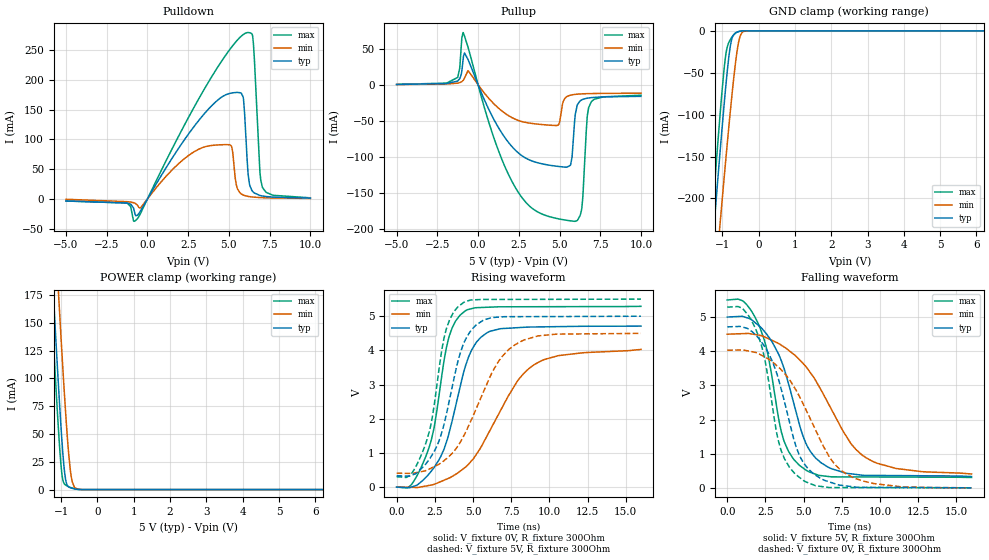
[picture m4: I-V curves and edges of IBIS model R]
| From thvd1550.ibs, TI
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|   R Model
[Model]   R
Model_type   3-state
Polarity   Non-Inverting
Vmeas = 2.5
Vref = 0
Cref = 2pF
Rref = 100000
|   typ   min   max
C_comp   6.849E-12   6.632E-12   7.073E-12
| Where Nom  PVT is Nominal Process, 5V, 27C
|   Fast PVT is Strong Process,  5.5V, -40C
|   Slow PVT is Weak Process,   4.5, 150C
[Voltage Range]   5   4.5   5.5
|Junction Temperature
[Temperature Range]   27   150   -40
[Pullup Reference]   5   4.5   5.5
[Pulldown Reference]   -0   0   0
[Power Clamp Reference]   5   4.5   5.5
[GND Clamp Reference]   0   0   0
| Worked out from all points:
|   slope of the pulldown table from 0 to 0.75 V, typ, clamps not added: 21.5 ohm
|   slope of the pullup table from 0 to 0.75 V, typ, clamps not added: 19.6 ohm
|   GND clamp passes 1 mA (typ) near -0.56 V on its own axis
|   POWER clamp passes 1 mA (typ) near -0.67 V on its own axis
|   falling waveform, V_fixture 5V, R_fixture 300Ohm: 20-80 % time 2.01ns typ, 3.35ns min, 1.42ns max; typ from 5 V to 0.332 V
|   rising waveform, V_fixture 0V, R_fixture 300Ohm: 20-80 % time 1.74ns typ, 3.15ns min, 1.29ns max; typ from 0 V to 4.71 V
|   rising waveform, V_fixture 5V, R_fixture 300Ohm: 20-80 % time 1.58ns typ, 2.64ns min, 1.21ns max; typ from 0.332 V to 5 V
|   falling waveform, V_fixture 0V, R_fixture 300Ohm: 20-80 % time 1.85ns typ, 2.86ns min, 1.37ns max; typ from 4.71 V to 0 V
[Pulldown]
|   Voltage   I(typ)   I(min)   I(max)
-5V       -3.551mA   -659.8uA   -3.569mA
-1.25V    -6.955mA   -4.705mA   -6.847mA
-725mV    -28.39mA   -7.89mA    -36.18mA
4.825V    175.4mA    91.28mA    242.6mA
5.17V     178.1mA    87.48mA    255.5mA
5.455V    179mA      23.58mA    265.2mA
5.875V    171.4mA    6.552mA    276.4mA
6.175V    42.48mA    4.211mA    279.8mA
6.505V    11.16mA    3.008mA    260.7mA
6.895V    5.857mA    2.243mA    48.82mA
7.06V     4.87mA     2.024mA    19.45mA
10V       1.206mA    734uA      1.774mA
[GND Clamp]
|   Voltage   I(typ)   I(min)   I(max)
-5V       -2.38A     -2.296A    -2.499A
-1.445V   -353.1mA   -424.4mA   -321.7mA
-1.25V    -245.9mA   -325.1mA   -206.9mA
-1.13V    -181.3mA   -264.9mA   -138.3mA
-1.055V   -141.8mA   -227.7mA   -97.28mA
-905mV    -67.29mA   -154.9mA   -29.35mA
-815mV    -29.82mA   -112.9mA   -13.49mA
-740mV    -10.26mA   -79.67mA   -7.859mA
-560mV    -1mA       -15.84mA   -1.073mA
-455mV    -200.7uA   -2.147mA   -166.1uA
-230mV    -1.03uA    -16.12uA   -110.4nA
10V       0A         0A         0A
[Pullup]
|   Voltage   I(typ)   I(min)   I(max)
-5V       386.8uA    262.1uA    493.5uA
-1.25V    5.15mA     2.234mA    10.1mA
-920mV    34.53mA    5.961mA    72.32mA
2.305V    -91.04mA   -48.01mA   -143.1mA
4.915V    -113.2mA   -56.03mA   -185.8mA
5.455V    -114.3mA   -16.34mA   -187.9mA
5.77V     -100.4mA   -13.95mA   -188.9mA
5.92V     -52.47mA   -13.45mA   -189.3mA
6.37V     -20.94mA   -12.67mA   -171.3mA
6.7V      -18.66mA   -12.39mA   -45.1mA
6.955V    -17.86mA   -12.24mA   -23.47mA
10V       -16.06mA   -11.75mA   -14.54mA
[POWER Clamp]
|   Voltage   I(typ)   I(min)   I(max)
-5V       2.654A     2.729A     2.619A
-1.415V   301.7mA    386.9mA    260mA
-1.25V    199mA      284.5mA    157mA
-1.16V    144.6mA    229.7mA    103mA
-1.085V   101mA      185mA      60.66mA
-1.055V   84.24mA    167.4mA    45.13mA
-980mV    45.5mA     124.7mA    14.71mA
-875mV    8.975mA    69.22mA    4.05mA
-740mV    1.599mA    16.08mA    1.911mA
-635mV    710.3uA    2.214mA    791.3uA
-440mV    33.16uA    97.23uA    17.39uA
10V       0A         0A         0A
[Ramp]
R_load = 300
|   typ   min   max
dV/dt_r   2.82706/1.73801e-09   2.4158/3.13642e-09   3.17347/1.28911e-09
dV/dt_f   2.80087/1.99301e-09   2.45509/3.33064e-09   3.11776/1.41101e-09
[Falling Waveform]
V_fixture = 5V
V_fixture_min = 4.5V
V_fixture_max = 5.5V
R_fixture = 300Ohm
C_fixture = 0F
|   Time   V(typ)   V(min)   V(max)
0s        5V         4.498V     5.5V
1.013ns   5.019V     4.515V     5.476V
1.816ns   4.841V     4.489V     5.004V
2.447ns   4.575V     4.418V     4.298V
2.938ns   4.273V     4.317V     3.23V
3.751ns   3.455V     4.116V     1.335V
5.163ns   1.294V     3.545V     517.2mV
6.561ns   618mV      2.521V     336.2mV
9.16ns    365.9mV    863.2mV    318.9mV
16ns      331.7mV    406.3mV    303.7mV
[Rising Waveform]
V_fixture = 0V
V_fixture_min = 0V
V_fixture_max = 0V
R_fixture = 300Ohm
C_fixture = 0F
|   Time   V(typ)   V(min)   V(max)
0s        471.2uV    1.853mV    91.22uV
785.7ps   -18.55mV   -6.369mV   -873.1uV
1.62ns    159.3mV    6.117mV    589.2mV
2.28ns    473mV      60.99mV    1.394V
2.784ns   807.7mV    140.9mV    2.705V
3.456ns   1.62V      267mV      4.432V
4.471ns   3.485V     569mV      5.15V
5.929ns   4.518V     1.505V     5.262V
9.072ns   4.685V     3.599V     5.278V
16ns      4.712V     4.028V     5.289V
[Rising Waveform]
V_fixture = 5V
V_fixture_min = 4.5V
V_fixture_max = 5.5V
R_fixture = 300Ohm
C_fixture = 0F
|   Time   V(typ)   V(min)   V(max)
0s        331.7mV    406.3mV    303.7mV
864.4ps   327.1mV    401.2mV    338.4mV
1.442ns   467.9mV    436.8mV    763.3mV
2.139ns   812.2mV    528.4mV    1.623V
2.552ns   1.122V     620.4mV    2.697V
3.279ns   2.172V     834.6mV    4.663V
4.389ns   4.2V       1.495V     5.403V
5.63ns    4.871V     2.728V     5.491V
7.724ns   4.987V     4.156V     5.492V
16ns      5V         4.498V     5.5V
[Falling Waveform]
|Gnd
V_fixture = 0V
V_fixture_min = 0V
V_fixture_max = 0V
R_fixture = 300Ohm
C_fixture = 0F
|   Time   V(typ)   V(min)   V(max)
0s        4.712V     4.028V     5.289V
1.442ns   4.634V     4.001V     5.011V
2.08ns    4.367V     3.921V     4.397V
2.641ns   3.995V     3.789V     3.313V
3.52ns    2.916V     3.464V     1.11V
4.39ns    1.381V     2.945V     438.2mV
5.002ns   730.4mV    2.43V      212.8mV
6.766ns   162.6mV    851.5mV    9.236mV
8.202ns   32.95mV    312.4mV    8.244mV
16ns      470.4uV    1.853mV    91.26uV
